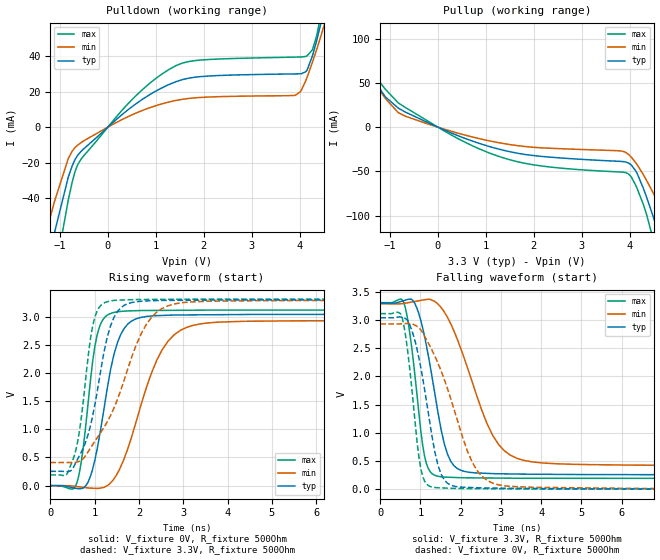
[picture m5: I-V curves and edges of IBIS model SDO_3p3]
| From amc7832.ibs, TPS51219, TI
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|   Model
[Model]   SDO_3p3
Model_type   Output
Polarity   Non-Inverting
Vmeas = 1.65
Vref = 0
Cref = 1pF
Rref = 100000
|   typ   min   max
C_comp   1pF   1pF   1pF
[Voltage Range]   3.3   3.29   3.31
[Temperature Range]   27   125   -40
[Pullup Reference]   3.3   3.29   3.31
[Pulldown Reference]   -0   -0   -0
[Power Clamp Reference]   3.3   3.29   3.31
[GND Clamp Reference]   -0   -0   -0
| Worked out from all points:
|   slope of the pulldown table from 0 to 0.495 V, typ, clamps not added: 43.7 ohm
|   slope of the pullup table from 0 to 0.495 V, typ, clamps not added: 44.1 ohm
|   falling waveform, V_fixture 3.3V, R_fixture 500Ohm: 20-80 % time 467ps typ, 890ps min, 298ps max; typ from 3.3 V to 0.254 V
|   rising waveform, V_fixture 0V, R_fixture 500Ohm: 20-80 % time 430ps typ, 764ps min, 277ps max; typ from 0 V to 3.04 V
|   rising waveform, V_fixture 3.3V, R_fixture 500Ohm: 20-80 % time 471ps typ, 891ps min, 298ps max; typ from 0.254 V to 3.3 V
|   falling waveform, V_fixture 0V, R_fixture 500Ohm: 20-80 % time 444ps typ, 854ps min, 278ps max; typ from 3.04 V to 0 V
[Pulldown]
|   Voltage   I(typ)   I(min)   I(max)
-3.3V     -462mA     -322.2mA   -598.2mA
-1.379V   -101.9mA   -70.08mA   -135.8mA
-1.112V   -59.46mA   -41.8mA    -84.03mA
-825mV    -28.1mA    -17.68mA   -41.05mA
-627mV    -15.77mA   -10.07mA   -21.05mA
511.5mV   11.65mA    7.022mA    15.7mA
1.422V    25.6mA     15.04mA    34.63mA
3.907V    29.96mA    17.95mA    39.41mA
4.155V    32.26mA    28.18mA    40.19mA
4.372V    50.83mA    45.35mA    54.01mA
4.996V    121.8mA    99.73mA    143.2mA
6.59V     242.5mA    198.2mA    284.8mA
[Pullup]
|   Voltage   I(typ)   I(min)   I(max)
-3.3V     213mA      180.5mA    246.3mA
-2.26V    148.7mA    125.7mA    174.4mA
-1.874V   114mA      97.58mA    133.4mA
-1.171V   40.08mA    38.44mA    48.1mA
-646.8mV  16.21mA    11.77mA    21.2mA
1.393V    -26.43mA   -18.72mA   -35.13mA
3.967V    -40.29mA   -30.47mA   -52.57mA
4.155V    -52.4mA    -42.49mA   -69.41mA
4.471V    -98.27mA   -72.42mA   -123.3mA
4.61V     -121.6mA   -87.36mA   -154.6mA
5.046V    -199.5mA   -138.7mA   -258mA
6.59V     -494.3mA   -347.5mA   -634.2mA
[Ramp]
R_load = 500
|   typ   min   max
dV/dt_r   1.82528/4.29504e-10   1.75951/7.64353e-10   1.86931/2.76543e-10
dV/dt_f   1.82788/4.67166e-10   1.72803/8.89861e-10   1.87171/2.97888e-10
[Falling Waveform]
V_fixture = 3.3V
V_fixture_min = 3.29V
V_fixture_max = 3.31V
R_fixture = 500Ohm
C_fixture = 0F
|   Time   V(typ)   V(min)   V(max)
0s        3.3V       3.29V      3.31V
600ps     3.349V     3.298V     3.281V
850.4ps   3.306V     3.33V      2.093V
1.1ns     2.712V     3.362V     590.8mV
1.415ns   1.445V     3.298V     232.1mV
1.672ns   621.6mV    3.048V     211.9mV
1.905ns   370.8mV    2.678V     206mV
2.8ns     275.8mV    949.8mV    197.5mV
3.575ns   266.7mV    510.1mV    193mV
20ns      253.5mV    409.9mV    190.5mV
[Rising Waveform]
V_fixture = 0V
V_fixture_min = 0V
V_fixture_max = 0V
R_fixture = 500Ohm
C_fixture = 0F
|   Time   V(typ)   V(min)   V(max)
0s        153.5nV    -2.086uV   -17.33nV
576.1ps   -48.58mV   -14.53mV   2.894mV
708.9ps   -51.74mV   -27.13mV   473.8mV
850.4ps   60.56mV    -40.56mV   1.442V
1.1ns     833.9mV    -48.07mV   2.795V
1.501ns   2.498V     199.5mV    3.083V
1.827ns   2.916V     847.2mV    3.101V
2.515ns   3.019V     2.399V     3.109V
3.401ns   3.03V      2.871V     3.113V
20ns      3.042V     2.933V     3.116V
[Rising Waveform]
V_fixture = 3.3V
V_fixture_min = 3.29V
V_fixture_max = 3.31V
R_fixture = 500Ohm
C_fixture = 0F
|   Time   V(typ)   V(min)   V(max)
0s        253.5mV    409.7mV    190.5mV
496.3ps   293.2mV    410.1mV    429.7mV
634.2ps   496.7mV    425.4mV    854.1mV
779.7ps   736mV      513.5mV    1.751V
1.007ns   1.437V     787.7mV    2.992V
1.345ns   2.797V     1.222V     3.275V
1.594ns   3.157V     1.702V     3.293V
2.171ns   3.277V     2.866V     3.303V
2.942ns   3.288V     3.243V     3.307V
20ns      3.3V       3.29V      3.31V
[Falling Waveform]
|Gnd
V_fixture = 0V
V_fixture_min = 0V
V_fixture_max = 0V
R_fixture = 500Ohm
C_fixture = 0F
|   Time   V(typ)   V(min)   V(max)
0s        3.042V     2.933V     3.116V
533.6ps   3.055V     2.935V     3.072V
744.3ps   2.896V     2.938V     2.061V
1.007ns   2.162V     2.827V     367.4mV
1.288ns   932.9mV    2.464V     37.92mV
1.438ns   418.5mV    2.23V      24.53mV
1.672ns   105.3mV    1.783V     18.32mV
2.286ns   28.7mV     481.3mV    9.853mV
2.942ns   18.66mV    76.46mV    6.025mV
20ns      -17.62uV   268.1uV    577.4nV
